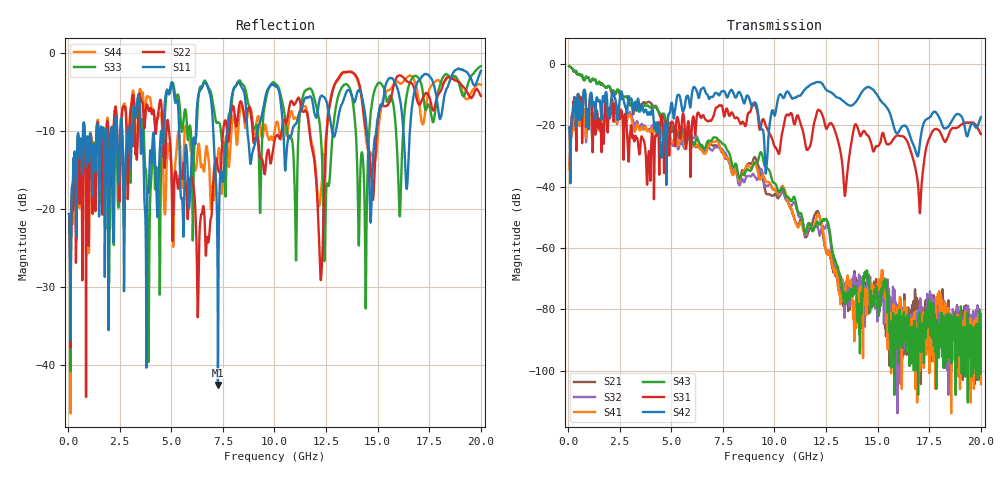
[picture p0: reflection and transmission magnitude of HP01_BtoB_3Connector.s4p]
# MHz S MA R 50.00
! FREQ  S11  S12  S13  S14
!  S21  S22  S23  S24
!  S31  S32  S33  S34
!  S41  S42  S43  S44
!  MAG  ANG  MAG  ANG  MAG  ANG  MAG  ANG
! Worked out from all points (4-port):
!   1996 points, 50 MHz to 20 GHz, reference 50 ohm
!   strongest paths, dB at 50 MHz, 5.04 GHz, 10.03 GHz, 15.02 GHz, 20 GHz:
!     S42: -20.7, -12.9, -16.5, -10.5, -17.3
!     S31: -20.7, -18.7, -27.2, -26.7, -22.8
!     S43: -0.6, -20.9, -39.0, -77.6, -100.9
!     S41: -34.0, -25.5, -40.9, -73.6, -104.4
!     S32: -34.0, -26.4, -41.1, -78.6, -81.6
!     S21: -0.6, -22.0, -42.5, -80.1, -83.2
!   lowest |S11| = -42.6 dB at 7.26 GHz (marker M1), VSWR 1.01, Z = 49.7 - j0.695 ohm
!   |S11| at or under -10 dB: start of sweep to 723.5 MHz; 3.61 GHz to 4.63 GHz (1.02 GHz wide, 24.8 % of centre); 5.379 GHz to 6.195 GHz (816.4 MHz wide, 14.1 % of centre)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
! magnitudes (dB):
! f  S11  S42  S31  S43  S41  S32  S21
! 50 MHz  -20.7  -20.7  -20.7  -0.6  -34.0  -34.0  -0.6
! 7.26 GHz  -42.6  -9.8  -13.9  -24.5  -25.3  -27.2  -27.0
! 9.6 GHz  -5.2  -34.6  -20.4  -33.6  -38.2  -39.6  -42.2
! 12.25 GHz  -5.5  -6.0  -15.6  -51.9  -51.2  -54.8  -51.6
! 13.87 GHz  -6.3  -12.8  -20.3  -72.8  -90.5  -69.6  -67.6
! 17.04 GHz  -3.4  -26.1  -48.6  -86.9  -88.4  -80.4  -94.9
! 20 GHz  -2.3  -17.3  -22.8  -100.9  -104.4  -81.6  -83.2
